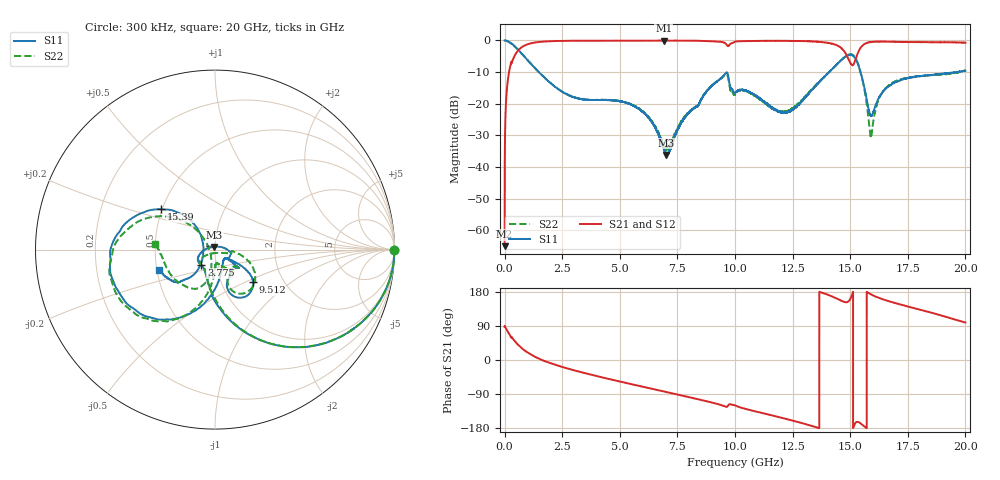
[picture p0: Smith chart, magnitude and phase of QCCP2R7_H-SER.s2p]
!{QCCP2R7}
!Johanson Technology Inc.
!www.johansontechnology.com
!Test Board Conditions:
!Substrate Type  RO4350B
!Substrate Thickness  20 mil
!Substrate Dk  3.66
!TL Type: GCPW
!TL Trace Width  36 mil
!TL Gap  12 mil
!Electrode orientation  Horizontal
!DUT TOPOLOGY	SERIES
!Mounting Pad LxW  26x36 mil
! Created Sat Jan  9 18:28:14 2021
# hz S ma R 50
! 2 Port Network Data from SP1.SP block
! freq  magS11  angS11  magS21  angS21  magS12  angS12  magS22  angS22
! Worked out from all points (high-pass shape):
!   20001 points, 300 kHz to 20 GHz, reference 50 ohm
!   highest |S21| = -0.03 dB at 6.906 GHz (marker M1); lowest = -65.0 dB at 300 kHz (marker M2)
!   |S21| within 3 dB of the highest: 603.5 MHz to 14.7 GHz (14.1 GHz wide, 184 % of centre); 15.39 GHz to end of sweep
!   lowest |S11| = -36.2 dB at 7.019 GHz (marker M3), VSWR 1.03, Z = 49.6 + j1.51 ohm
!   |S11| at or under -10 dB: 1.485 GHz to 14.08 GHz (12.6 GHz wide, 162 % of centre); 15.45 GHz to 19.58 GHz (4.125 GHz wide, 23.6 % of centre); 19.62163 GHz to 19.63457 GHz (12.95 MHz wide, 0.066 % of centre)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
!   |S22| runs from -34.5 to 0.0 dB; largest |S21 - S12| = 0.016
!   S11 on the Smith chart (normalised r, x): 300 kHz: open; 3.775 GHz: 0.85, -0.15; 9.512 GHz: 1.41, -0.56; 15.39 GHz: 0.49, +0.26; 20 GHz: 0.51, -0.13
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300000  0.9992 -0.2  0.0005621 87.1  0.0004637 92.8  0.9991 -0.2
1.263e8  0.9757 -13.7  0.2142 76.0  0.215 76.0  0.9753 -13.7
4.493e8  0.8035 -40.4  0.588 49.2  0.5897 49.3  0.8032 -40.3
1.3973e9  0.3407 -84.3  0.9363 6.1  0.9368 6.1  0.3413 -83.0
3.3343e9  0.1184 -124.3  0.9891 -32.3  0.9886 -32.3  0.1187 -119.6
3.7753e9  0.1149 -131.8  0.9902 -39.1  0.99 -39.0  0.1147 -125.3
5.6043e9  0.09298 -161.3  0.9911 -65.2  0.9903 -65.2  0.09407 -147.0
6.6673e9  0.03346 162.5  0.9946 -79.7  0.9946 -79.6  0.0355 -137.8
6.9063e9  0.01954 133.1  0.9965 -82.9  0.9948 -83.0  0.02258 -114.4
7.0193e9  0.01557 103.1  0.994 -84.5  0.9945 -84.5  0.01934 -90.7
7.8353e9  0.06142 3.8  0.9918 -95.7  0.9926 -95.7  0.06236 -17.8
9.5123e9  0.2796 -40.5  0.9302 -121.5  0.9309 -121.3  0.273 -35.1
1.00003e10  0.1486 -45.2  0.9533 -120.0  0.9533 -119.9  0.1399 -41.1
1.21753e10  0.0729 -44.0  0.9851 -154.9  0.9878 -154.8  0.07572 -85.9
1.33343e10  0.1645 -81.8  0.9656 -174.0  0.9702 -174.0  0.1681 -94.1
1.46733e10  0.513 -131.7  0.7234 155.0  0.7247 154.8  0.5125 -128.9
1.50713e10  0.5868 -174.1  0.4099 170.1  0.4069 169.8  0.6014 -167.0
1.53883e10  0.374 143.2  0.6989 -164.7  0.6944 -164.8  0.3795 151.0
1.58953e10  0.06448 176.0  0.9425 173.4  0.9434 173.4  0.03045 -161.9
1.62363e10  0.1224 -132.7  0.9585 164.1  0.9593 164.1  0.1155 -101.5
1.66673e10  0.1885 -130.7  0.9549 155.3  0.9537 155.2  0.1948 -106.7
2e10  0.3314 -160.0  0.9206 98.8  0.9129 98.6  0.3372 174.2
